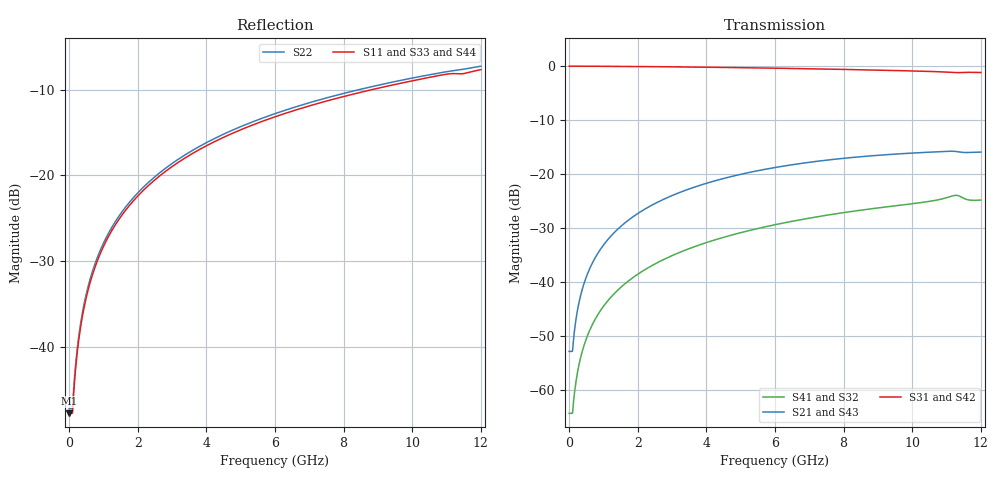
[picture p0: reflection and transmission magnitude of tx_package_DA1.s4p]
! Created Mon Sep 08 15:29:33 2014
# hz S db R 50
! 4 Port Network Data from SP1.SP block
! freq  dbS11  angS11  dbS12  angS12  dbS13  angS13  dbS14  angS14
!  dbS21  angS21  dbS22  angS22  dbS23  angS23  dbS24  angS24
!  dbS31  angS31  dbS32  angS32  dbS33  angS33  dbS34  angS34
!  dbS41  angS41  dbS42  angS42  dbS43  angS43  dbS44  angS44
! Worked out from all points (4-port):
!   1201 points, 1 MHz to 12 GHz, reference 50 ohm
!   strongest paths, dB at 1 MHz, 3.001 GHz, 6.001 GHz, 9.001 GHz, 12 GHz:
!     S31: 0.0, -0.1, -0.4, -0.7, -1.2
!     S42: 0.0, -0.2, -0.4, -0.8, -1.3
!     S21: -52.8, -24.0, -18.8, -16.5, -15.9
!     S43: -52.8, -24.0, -19.0, -16.8, -15.9
!     S41: -64.3, -35.1, -29.4, -26.3, -24.8
!     S32: -64.3, -35.1, -29.4, -26.4, -24.8
!   lowest |S11| = -47.8 dB at 1 MHz (marker M1), VSWR 1.01, Z = 50.1 + j0.388 ohm
!   |S11| at or under -10 dB: start of sweep to 8.812 GHz
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1000000  -47.79 71.4  -52.85 85.7  -0.01 -0.6  -64.32 -101.0
         -52.85 85.7  -47.24 68.9  -64.33 -100.6  -0.01 -0.7
         -0.01 -0.6  -64.33 -100.6  -47.79 70.8  -52.84 85.8
         -64.32 -101.0  -0.01 -0.7  -52.84 85.8  -47.24 68.3
9.1e7  -47.79 71.4  -52.85 85.7  -0.01 -0.6  -64.32 -101.0
       -52.85 85.7  -47.24 68.9  -64.33 -100.6  -0.01 -0.7
       -0.01 -0.6  -64.33 -100.6  -47.79 70.8  -52.84 85.8
       -64.32 -101.0  -0.01 -0.7  -52.84 85.8  -47.24 68.3
3.91e8  -36.39 83.5  -41.19 85.5  -0.02 -2.5  -52.67 -97.9
        -41.19 85.5  -35.98 82.6  -52.64 -97.8  -0.02 -2.7
        -0.02 -2.5  -52.64 -97.8  -36.38 81.2  -41.19 85.7
        -52.67 -97.9  -0.02 -2.7  -41.19 85.7  -35.98 80.2
8.21e8  -30.00 84.2  -34.85 82.7  -0.03 -5.2  -46.22 -102.9
        -34.85 82.7  -29.61 83.4  -46.20 -102.7  -0.04 -5.6
        -0.03 -5.2  -46.20 -102.7  -30.01 79.3  -34.84 83.1
        -46.22 -102.9  -0.04 -5.6  -34.84 83.1  -29.62 78.4
2.661e9  -19.99 79.4  -24.96 69.7  -0.12 -16.4  -36.12 -128.4
         -24.96 69.7  -19.63 78.2  -36.13 -127.6  -0.13 -17.7
         -0.12 -16.4  -36.13 -127.6  -20.02 64.1  -24.99 71.1
         -36.12 -128.4  -0.13 -17.7  -24.99 71.1  -19.66 62.2
6.491e9  -12.51 67.7  -18.28 43.2  -0.44 -39.4  -28.76 179.2
         -18.28 43.2  -12.14 64.9  -28.79 -179.2  -0.48 -42.3
         -0.44 -39.4  -28.79 -179.2  -12.58 31.1  -18.52 48.2
         -28.76 179.2  -0.48 -42.3  -18.52 48.2  -12.21 27.5
1.2e10  -7.65 50.9  -15.93 7.1  -1.18 -70.6  -24.81 106.2
        -15.93 7.1  -7.25 45.1  -24.82 108.8  -1.30 -75.9
        -1.18 -70.6  -24.82 108.8  -7.93 -13.3  -15.90 25.8
        -24.81 106.2  -1.30 -75.9  -15.90 25.8  -7.49 -17.8
